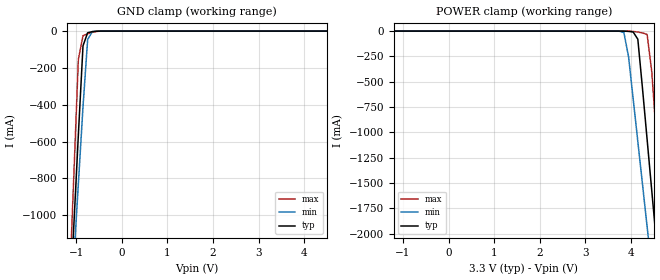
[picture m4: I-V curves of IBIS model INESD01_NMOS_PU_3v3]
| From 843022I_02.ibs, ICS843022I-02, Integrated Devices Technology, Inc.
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[Model] INESD01_NMOS_PU_3v3
Model_type   Input
Polarity   Non-Inverting
Vinl = 0.7V
Vinh = 1.3V
|   typ   min   max
C_comp   2pF   1.5pF   2.5pF
|   typ   min   max
[Voltage range]  3.3V   3.15V   3.45V
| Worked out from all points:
|   GND clamp passes 1 mA (typ) near -0.56 V on its own axis
[GND_clamp]
|Voltage   I(typ)   I(min)   I(max)
-3.3V     -12.24A    -10.56A    -15.06A
-1.157V   -1.578A    -1.673A    -1.45A
-1.055V   -1.071A    -1.251A    -801.8mA
-952.6mV  -564.4mA   -830.8mA   -154mA
-850.5mV  -79.92mA   -410.9mA   -24.97mA
-748.5mV  -8.956mA   -45.87mA   -14.66mA
-646.4mV  -3.019mA   -2.828mA   -6.626mA
-544.3mV  -652uA     -309.6uA   -1.636mA
6.6V      4.435nA    6.865nA    1.283nA
[POWER_clamp]
|Voltage   I(typ)   I(min)   I(max)
-3.3V     4.435nA    5.64nA     1.609nA
3.64V     -5.052uA   -135.1uA   -13.25nA
3.844V    -652uA     -14.51mA   -32.02uA
3.946V    -3.019mA   -250.2mA   -451.4uA
4.048V    -8.956mA   -669.7mA   -3.083mA
4.151V    -79.92mA   -1.09A     -9.442mA
4.355V    -1.071A    -1.933A    -33.35mA
4.457V    -1.578A    -2.355A    -402.1mA
4.559V    -2.085A    -2.777A    -1.05A
4.661V    -2.593A    -3.199A    -1.698A
4.763V    -3.101A    -3.622A    -2.347A
6.6V      -12.24A    -11.24A    -14.01A
